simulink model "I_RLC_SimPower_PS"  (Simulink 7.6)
settings: Solver=ode15s  StartTime=0.0  StopTime=0.14  RelTol=1e-3
PreLoadFcn:
  | clc
InitFcn:
  | R=1;
  | L=0.01;
  | C=1e-3;
StopFcn:
  | close all
  | load I_RLC_SimPower_PS.mat
  | plot(x(1,:),x(2,:))
  | hold on
  | plot(x(1,:),x(3,:))
  | plot(x(1,:),x(4,:))
  | %axis([0 0.14 -0.2 2.2])
  | grid
  | title('Courant dans le circuit RLC, tension aux bornes de C et échelon d''entrée')
  | xlabel('Circuit RLC - Simulation de la capacité et de l''inductance')
libraries: powerlib x7

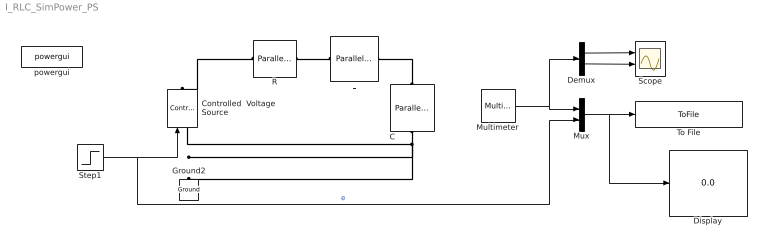
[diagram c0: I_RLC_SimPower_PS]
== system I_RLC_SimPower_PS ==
  C : powerlib/Elements/Parallel RLC Branch  DialogController=POWERSYS.PowerSysDialog  PhysicalDomain=powersysdomain  SubClassName=unknown  LeftPortType=p1  RightPortType=p1  LConnTagsString=a  RConnTagsString=__new0  BranchType=C  Resistance=1  Inductance=1e-3  SetiL0=off  InitialCurrent=0  Capacitance=C  Setx0=off  InitialVoltage=0  Measurements=Branch voltage and current
  Controlled  Voltage Source : powerlib/Electrical Sources/Controlled Voltage Source  DialogController=POWERSYS.PowerSysDialog  SystemSampleTime=-1  Initialize=on  Source_Type=AC  Amplitude=0  Phase=0  Frequency=0  Measurements=None
  Demux : Demux  Outputs=2
  Display : Display
  Ground2 : powerlib/Elements/Ground  DialogController=POWERSYS.PowerSysDialog  PhysicalDomain=powersysdomain  SubClassName=unknown  LeftPortType=p1  RightPortType=p1  LConnTagsString=a
  L : powerlib/Elements/Parallel RLC Branch  DialogController=POWERSYS.PowerSysDialog  PhysicalDomain=powersysdomain  SubClassName=unknown  LeftPortType=p1  RightPortType=p1  LConnTagsString=a  RConnTagsString=__new0  BranchType=L  Resistance=1  Inductance=L  SetiL0=off  InitialCurrent=0  Capacitance=1e-6  Setx0=off  InitialVoltage=0  Measurements=None
  Multimeter : powerlib/Measurements/Multimeter  SystemSampleTime=-1  PhasorSimulation=off  OutputType=Complex  sel=[1 2]  L=2  Gain=[1 1]  yselected={'Ub: C','Ib: C'};  PSBOutputType=1  PSBequivalent=0  AxesSetting=[0,0.1,-100,100]  Display=0  SavedBlockNames=-11
  Mux : Mux  Inputs=2
  R : powerlib/Elements/Parallel RLC Branch  DialogController=POWERSYS.PowerSysDialog  PhysicalDomain=powersysdomain  SubClassName=unknown  LeftPortType=p1  RightPortType=p1  LConnTagsString=a  RConnTagsString=__new0  BranchType=R  Resistance=R  Inductance=10e-03  SetiL0=off  InitialCurrent=0  Capacitance=[]  Setx0=off  InitialVoltage=0  Measurements=None
  Scope : Scope  NumInputPorts=2
  Step1 : Step  Time=0.02  SampleTime=0
  To File : ToFile  Filename=I_RLC_SimPower_PS  MatrixName=x
  powergui : powerlib/powergui  SystemSampleTime=-1  SimulationMode=Continuous  SampleTime=0  frequency=60  SPID=off  DisableSnubberDevices=off  DisableRonSwitches=off  DisableVfSwitches=off  SwTol=0  Interpol=off  frequencyindice=0  echomessages=off  HookPort=off  DisplayEquations=off  FunctionMessages=off  EnableUseOfTLC=off  x0status=blocks  RestoreLinks=warning  ResistiveCurrentMeasurement=off  Frange=[0:2:500]  Ylog=off  Xlog=on  ShowGrid=on  save=off  variable=ZData  ZoomFFT=on  StartTime=0.0  cycles=1  DisplayStyle=1  fundamental=60  FreqAxis=off  MaxFrequency=1000  frequencyindicesteady=60  RmsSteady=1  display=off  Ts=0  methode=off
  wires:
  Step1/1 -> Controlled  Voltage Source/1, Mux/2  "e"
  Multimeter/1 -> Demux/1, Mux/1
  Demux/1 -> Scope/1
  Demux/2 -> Scope/2
  Mux/1 -> To File/1, Display/1
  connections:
  R/RConn1 -- Controlled  Voltage Source/RConn1
  R/LConn1 -- L/LConn1
  C/LConn1 -- L/RConn1
  C/RConn1 -- Controlled  Voltage Source/LConn1 -- Ground2/LConn1
